DATA_BLOCK "FDB_DP_CMD"
TITLE =
VERSION : 0.1
NON_RETAIN


  STRUCT
   cPLC_OK : BOOL ;	//Trvale Log.1 - test komunikace s PLC
   cBLOKADY_OK : BOOL ;	//Splnìny blokády provozu kotle
   cHORI_UHLI : BOOL ;	//Provoz uhelných hoøákù
   Bit0_03 : BOOL ;
   Bit0_04 : BOOL ;
   Bit0_05 : BOOL ;
   Bit0_06 : BOOL ;
   cACK_ALL : BOOL ;	//Kvitace celková pro všechny hoøáky
   cSTART_H1 : BOOL ;	//Start/Stop hoøáku H1
   Bit1_01 : BOOL ;
   Bit1_02 : BOOL ;
   Bit1_03 : BOOL ;
   Bit1_04 : BOOL ;
   Bit1_05 : BOOL ;
   Bit1_06 : BOOL ;
   cACK_H1 : BOOL ;	//Kvitace hoøáku H1
   cSTART_H2 : BOOL ;	//Start/Stop hoøáku H2
   Bit2_01 : BOOL ;
   Bit2_02 : BOOL ;
   Bit2_03 : BOOL ;
   Bit2_04 : BOOL ;
   Bit2_05 : BOOL ;
   Bit2_06 : BOOL ;
   cACK_H2 : BOOL ;	//Kvitace hoøáku H2
   cSTART_H3 : BOOL ;	//Start/Stop hoøáku H3
   Bit3_01 : BOOL ;
   Bit3_02 : BOOL ;
   Bit3_03 : BOOL ;
   Bit3_04 : BOOL ;
   Bit3_05 : BOOL ;
   Bit3_06 : BOOL ;
   cACK_H3 : BOOL ;	//Kvitace hoøáku H2
   cSTART_H4 : BOOL ;	//Start/Stop hoøáku H4
   Bit4_01 : BOOL ;
   Bit4_02 : BOOL ;
   Bit4_03 : BOOL ;
   Bit4_04 : BOOL ;
   Bit4_05 : BOOL ;
   Bit4_06 : BOOL ;
   cACK_H4 : BOOL ;	//Kvitace hoøáku H4
   W6 : WORD ;
   cSP_H1 : INT ;	//Žádaný výkon hoøáku H1 [0..10000]=[0..100%]
   cSP_H2 : INT ;	//Žádaný výkon hoøáku H2 [0..10000]=[0..100%]
   cSP_H3 : INT ;	//Žádaný výkon hoøáku H3 [0..10000]=[0..100%]
   cSP_H4 : INT ;	//Žádaný výkon hoøáku H4 [0..10000]=[0..100%]
  END_STRUCT ;
BEGIN
   cPLC_OK := FALSE;
   cBLOKADY_OK := FALSE;
   cHORI_UHLI := FALSE;
   Bit0_03 := FALSE;
   Bit0_04 := FALSE;
   Bit0_05 := FALSE;
   Bit0_06 := FALSE;
   cACK_ALL := FALSE;
   cSTART_H1 := FALSE;
   Bit1_01 := FALSE;
   Bit1_02 := FALSE;
   Bit1_03 := FALSE;
   Bit1_04 := FALSE;
   Bit1_05 := FALSE;
   Bit1_06 := FALSE;
   cACK_H1 := FALSE;
   cSTART_H2 := FALSE;
   Bit2_01 := FALSE;
   Bit2_02 := FALSE;
   Bit2_03 := FALSE;
   Bit2_04 := FALSE;
   Bit2_05 := FALSE;
   Bit2_06 := FALSE;
   cACK_H2 := FALSE;
   cSTART_H3 := FALSE;
   Bit3_01 := FALSE;
   Bit3_02 := FALSE;
   Bit3_03 := FALSE;
   Bit3_04 := FALSE;
   Bit3_05 := FALSE;
   Bit3_06 := FALSE;
   cACK_H3 := FALSE;
   cSTART_H4 := FALSE;
   Bit4_01 := FALSE;
   Bit4_02 := FALSE;
   Bit4_03 := FALSE;
   Bit4_04 := FALSE;
   Bit4_05 := FALSE;
   Bit4_06 := FALSE;
   cACK_H4 := FALSE;
   W6 := W#16#0;
   cSP_H1 := 0;
   cSP_H2 := 0;
   cSP_H3 := 0;
   cSP_H4 := 0;
END_DATA_BLOCK

DATA_BLOCK "FDB_DP_STATE"
TITLE =
VERSION : 0.1
NON_RETAIN


  STRUCT
   sPLC_OK : BOOL ;	//Trvale Log.1 - test komunikace s PLC
   sSYSTEM_OK : BOOL ;	//Systém pøipraven (STOP tl., napájení, HW)
   Bit0_02 : BOOL ;
   Bit0_03 : BOOL ;
   sERROR_Hx : BOOL ;	//Spoleèná porucha hoøákù (technologická)
   sSAFE_ERR : BOOL ;	//Porucha SAFETY I/O PLC
   Bit0_06 : BOOL ;
   sACK_REQ : BOOL ;	//Systém vyžaduje kvitaci
   sPROVOZ_H1 : BOOL ;	//Provoz hoøáku H1
   sREADY_H1 : BOOL ;	//Hoøák pøipraven H1 (STOP tl., napájení, HW)
   sSTART_H1 : BOOL ;	//Start hoøáku H1
   sLOCAL_H1 : BOOL ;	//Lokální øízení hoøáku H1
   sERROR_H1 : BOOL ;	//Porucha hoøáku H1 (technologická)
   sFERR_H1 : BOOL ;	//Porucha SAFETY I/O hoøáku H1
   Bit1_06 : BOOL ;
   sACK_REQ_H1 : BOOL ;	//Hoøák H1 vyžaduje kvitaci
   sPROVOZ_H2 : BOOL ;	//Provoz hoøáku H2
   sREADY_H2 : BOOL ;	//Hoøák pøipraven H2 (STOP tl., napájení, HW)
   sSTART_H2 : BOOL ;	//Start hoøáku H2
   sLOCAL_H2 : BOOL ;	//Lokální øízení hoøáku H2
   sERROR_H2 : BOOL ;	//Porucha hoøáku H2 (technologická)
   sFERR_H2 : BOOL ;	//Porucha SAFETY I/O hoøáku H2
   Bit2_06 : BOOL ;
   sACK_REQ_H2 : BOOL ;	//Hoøák H2 vyžaduje kvitaci
   sPROVOZ_H3 : BOOL ;	//Provoz hoøáku H3
   sREADY_H3 : BOOL ;	//Hoøák pøipraven H3 (STOP tl., napájení, HW)
   sSTART_H3 : BOOL ;	//Start hoøáku H3
   sLOCAL_H3 : BOOL ;	//Lokální øízení hoøáku H3
   sERROR_H3 : BOOL ;	//Porucha hoøáku H3 (technologická)
   sFERR_H3 : BOOL ;	//Porucha SAFETY I/O hoøáku H3
   Bit3_06 : BOOL ;
   sACK_REQ_H3 : BOOL ;	//Hoøák H3 vyžaduje kvitaci
   sPROVOZ_H4 : BOOL ;	//Provoz hoøáku H4
   sREADY_H4 : BOOL ;	//Hoøák pøipraven H4 (STOP tl., napájení, HW)
   sSTART_H4 : BOOL ;	//Start hoøáku H4
   sLOCAL_H4 : BOOL ;	//Lokální øízení hoøáku H4
   sERROR_H4 : BOOL ;	//Porucha hoøáku H4 (technologická)
   sFERR_H4 : BOOL ;	//Porucha SAFETY I/O hoøáku H4
   Bit4_06 : BOOL ;
   sACK_REQ_H4 : BOOL ;	//Hoøák H4 vyžaduje kvitaci
   W6 : WORD ;
   sSP_H1 : INT ;	//Výkon hoøáku H1 [0..10000]=[0..100%]
   sSP_H2 : INT ;	//Výkon hoøáku H2 [0..10000]=[0..100%]
   sSP_H3 : INT ;	//Výkon hoøáku H3 [0..10000]=[0..100%]
   sSP_H4 : INT ;	//Výkon hoøáku H4 [0..10000]=[0..100%]
   K04HJA10CR001XB01 : BOOL ;	//I0.0: HOØÁK È.1 - HLÍDAÈ PLAMENE - PLAMEN HOØÍ
   K04HJA20CR001XB01 : BOOL ;	//I0.1: HOØÁK È.2 - HLÍDAÈ PLAMENE - PLAMEN HOØÍ
   K04HJA30CR001XB01 : BOOL ;	//I0.2: HOØÁK È.3 - HLÍDAÈ PLAMENE - PLAMEN HOØÍ
   K04HJA40CR001XB01 : BOOL ;	//I0.3: HOØÁK È.4 - HLÍDAÈ PLAMENE - PLAMEN HOØÍ
   K04CJF21EA001XB01 : BOOL ;	//I0.4: NAPÁJENÍ HOØÁKU È.1 - OK
   K04CJF21EA001XB02 : BOOL ;	//I0.5: NAPÁJENÍ SERVOPOHONÙ HOØÁK 1 - OK
   K04HHA20AV11XG10 : BOOL ;	//I0.6: HOØÁK È.1 - STYKAÈE BEZP. VYPNUTÍ ROZEPNUTY (PØIPRAVENY)
   K04CJF21EA001XB03 : BOOL ;	//I0.7: NAPÁJENÍ HOØÁKU È.2 - OK
   K04CJF21EA001XB04 : BOOL ;	//I1.0: NAPÁJENÍ SERVOPOHONÙ HOØÁK 2 - OK
   K04HHA20AV21XG10 : BOOL ;	//I1.1: HOØÁK È.2 - STYKAÈE BEZP. VYPNUTÍ ROZEPNUTY (PØIPRAVENY)
   K04CJF21EA001XB05 : BOOL ;	//I1.2: NAPÁJENÍ HOØÁKU È.3 - OK
   K04CJF21EA001XB06 : BOOL ;	//I1.3: NAPÁJENÍ SERVOPOHONÙ HOØÁK 3 - OK
   K04HHA20AV31XG10 : BOOL ;	//I1.4: HOØÁK È.3 - STYKAÈE BEZP. VYPNUTÍ ROZEPNUTY (PØIPRAVENY)
   K04CJF21EA001XB07 : BOOL ;	//I1.5: NAPÁJENÍ HOØÁKU È.4 - OK
   K04CJF21EA001XB08 : BOOL ;	//I1.6: NAPÁJENÍ SERVOPOHONÙ HOØÁK 4 - OK
   K04HHA20AV41XG10 : BOOL ;	//I1.7: HOØÁK È.3 - STYKAÈE BEZP. VYPNUTÍ ROZEPNUTY (PØIPRAVENY)
   K04HJA10CR001XB51 : BOOL ;	//I100.0: HOØÁK È.1 - PLAMEN HOØÍ HLÍDAÈ PLAMENE (FAIL SAFE)
   K04HJA20CR001XB51 : BOOL ;	//I100.1: HOØÁK È.2 - PLAMEN HOØÍ HLÍDAÈ PLAMENE (FAIL SAFE)
   K04HJA30CR001XB51 : BOOL ;	//I100.2: HOØÁK È.3 - PLAMEN HOØÍ HLÍDAÈ PLAMENE (FAIL SAFE)
   K04HJA40CR001XB51 : BOOL ;	//I100.3: HOØÁK È.4 - PLAMEN HOØÍ HLÍDAÈ PLAMENE (FAIL SAFE)
   K04HHG36CP031XG01 : BOOL ;	//I100.4: HOØÁK 1 - TLAK PLYNU MIN - ZKOUŠKA TÌSNOSTI
   K04HHL11CP001XG01 : BOOL ;	//I100.5: HOØÁK 1 - TLAK SEKUNDÁRNÍHO VZDUCHU MIN
   K04HHA20AV011XB01 : BOOL ;	//I100.6: HOØÁK 1 - HOØÁK - ZAPALOVACÍ PLAMEN
   K04HHG37CP031XG01 : BOOL ;	//I100.7: HOØÁK 2 - TLAK PLYNU MIN - ZKOUŠKA TÌSNOSTI
   K04HHL71CP001XG01 : BOOL ;	//I101.0: HOØÁK 2 - TLAK SEKUNDÁRNÍHO VZDUCHU MIN
   K04HHA20AV021XB01 : BOOL ;	//I101.1: HOØÁK 2 - HOØÁK - ZAPALOVACÍ PLAMEN
   K04HHG38CP031XG01 : BOOL ;	//I101.2: HOØÁK 3 - TLAK PLYNU MIN - ZKOUŠKA TÌSNOSTI
   K04HHL51CP001XG01 : BOOL ;	//I101.3: HOØÁK 3 - TLAK SEKUNDÁRNÍHO VZDUCHU MIN
   K04HHA20AV031XB01 : BOOL ;	//I101.4: HOØÁK 3 - HOØÁK - ZAPALOVACÍ PLAMEN
   K04HHG39CP031XG01 : BOOL ;	//I101.5: HOØÁK 4 - TLAK PLYNU MIN - ZKOUŠKA TÌSNOSTI
   K04HHL31CP001XG01 : BOOL ;	//I101.6: HOØÁK 4 - TLAK SEKUNDÁRNÍHO VZDUCHU MIN
   K04HHA20AV041XB01 : BOOL ;	//I101.7: HOØÁK 4 - HOØÁK - ZAPALOVACÍ PLAMEN
   K04HHL11AS010XB51 : BOOL ;	//I102.0: HOØÁK È.1 - POLOHA KLAPKY VZDUCHU PRO ZAPALOVÁNÍ
   K04HHL11AS010XB53 : BOOL ;	//I102.1: HOØÁK È.1 - POLOHA KLAPKY VZDUCHU PRO PROFUK
   K04HHG36AS001XB51 : BOOL ;	//I102.2: HOØÁK È.1 - POLOHA KLAPKY PLYNU PRO ZAPALOVÁNÍ
   K04HHL71AS010XB51 : BOOL ;	//I102.3: HOØÁK È.2 - POLOHA KLAPKY VZDUCHU PRO ZAPALOVÁNÍ
   K04HHL71AS010XB53 : BOOL ;	//I102.4: HOØÁK È.2 - POLOHA KLAPKY VZDUCHU PRO PROFUK
   K04HHG37AS001XB51 : BOOL ;	//I102.5: HOØÁK È.2 - POLOHA KLAPKY PLYNU PRO ZAPALOVÁNÍ
   K04HHL51AS010XB51 : BOOL ;	//I102.6: HOØÁK È.3 - POLOHA KLAPKY VZDUCHU PRO ZAPALOVÁNÍ
   K04HHL51AS010XB53 : BOOL ;	//I102.7: HOØÁK È.3 - POLOHA KLAPKY VZDUCHU PRO PROFUK
   K04HHG38AS001XB51 : BOOL ;	//I110.0: HOØÁK È.3 - POLOHA KLAPKY PLYNU PRO ZAPALOVÁNÍ
   K04HHL31AS010XB51 : BOOL ;	//I110.1: HOØÁK È.4 - POLOHA KLAPKY VZDUCHU PRO ZAPALOVÁNÍ
   K04HHL31AS010XB53 : BOOL ;	//I110.2: HOØÁK È.4 - POLOHA KLAPKY VZDUCHU PRO PROFUK
   K04HHG39AS001XB51 : BOOL ;	//I110.3: HOØÁK È.4 - POLOHA KLAPKY PLYNU PRO ZAPALOVÁNÍ
   K04HHA20CH001YG11 : BOOL ;	//I110.4: TLAÈÍTKO BEZPEÈNOSTNÍ VYPNUTÍ - DVEØE ROZVADÌÈE
   K04HHA20CH001YG21 : BOOL ;	//I110.5: TLAÈÍTKO BEZPEÈNOSTNÍ VYPNUTÍ - OVLÁDACÍ SKØÍÒKA
   K04HHA20CH001YG31 : BOOL ;	//I110.6: TLAÈÍTKO BEZPEÈNOSTNÍ VYPNUTÍ - TLAÈÍTKO U DVEØÍ
   FI110_7 : BOOL ;	//I110.7: REZERVA
   K04HHG36CP001XG01 : BOOL ;	//I111.0: HOØÁK 1 - TLAK PLYNU MIN
   K04HHG36CP002XG01 : BOOL ;	//I111.1: HOØÁK 1 - TLAK PLYNU MAX
   K04HHG37CP001XG01 : BOOL ;	//I111.2: HOØÁK 2 - TLAK PLYNU MIN
   K04HHG37CP002XG01 : BOOL ;	//I111.3: HOØÁK 2 - TLAK PLYNU MAX
   K04HHG38CP001XG01 : BOOL ;	//I111.4: HOØÁK 3 - TLAK PLYNU MIN
   K04HHG38CP002XG01 : BOOL ;	//I111.5: HOØÁK 3 - TLAK PLYNU MAX
   K04HHG39CP001XG01 : BOOL ;	//I111.6: HOØÁK 4 - TLAK PLYNU MIN
   K04HHG39CP002XG01 : BOOL ;	//I111.7: HOØÁK 4 - TLAK PLYNU MAX
   FI112_0 : BOOL ;	//I112.0: REZERVA
   FI112_1 : BOOL ;	//I112.1: REZERVA
   FI112_2 : BOOL ;	//I112.2: REZERVA
   FI112_3 : BOOL ;	//I112.3: REZERVA
   FI112_4 : BOOL ;	//I112.4: REZERVA
   FI112_5 : BOOL ;	//I112.5: REZERVA
   FI112_6 : BOOL ;	//I112.6: REZERVA
   FI112_7 : BOOL ;	//I112.7: REZERVA
   K04HJA10CR001YB01 : BOOL ;	//Q0.0: HOØÁK 1 - UVOLNÌNÍ SNÍMAÈE PLAMENE
   K04HHL11AA101YB01 : BOOL ;	//Q0.1: HOØÁK 1 - TØÍCESTNÝ VENTIL SPAL. VZDUCHU - OTEVØÍT
   K04HJA20CR001YB01 : BOOL ;	//Q0.2: HOØÁK 2 - UVOLNÌNÍ SNÍMAÈE PLAMENE
   K04HHL71AA101YB01 : BOOL ;	//Q0.3: HOØÁK 2 - TØÍCESTNÝ VENTIL SPAL. VZDUCHU - OTEVØÍT
   K04HJA30CR001YB01 : BOOL ;	//Q0.4: HOØÁK 3 - UVOLNÌNÍ SNÍMAÈE PLAMENE
   K04HHL51AA101YB01 : BOOL ;	//Q0.5: HOØÁK 3 - TØÍCESTNÝ VENTIL SPAL. VZDUCHU - OTEVØÍT
   K04HJA40CR001YB01 : BOOL ;	//Q0.6: HOØÁK 4 - UVOLNÌNÍ SNÍMAÈE PLAMENE
   K04HHL31AA101YB01 : BOOL ;	//Q0.7: HOØÁK 4 - TØÍCESTNÝ VENTIL SPAL. VZDUCHU - OTEVØÍT
   Q1_0 : BOOL ;	//Q1.0: REZERVA
   Q1_1 : BOOL ;	//Q1.1: REZERVA
   Q1_2 : BOOL ;	//Q1.2: REZERVA
   Q1_3 : BOOL ;	//Q1.3: REZERVA
   Q1_4 : BOOL ;	//Q1.4: REZERVA
   Q1_5 : BOOL ;	//Q1.5: REZERVA
   Q1_6 : BOOL ;	//Q1.6: REZERVA
   Q1_7 : BOOL ;	//Q1.7: REZERVA
   K04HHA20AV011YB03 : BOOL ;	//Q200.0: VYPNUTÍ HOØÁKU 1 - FAIL SAFE
   K04HHG36AA101YB01 : BOOL ;	//Q200.1: HOØÁK 1 - PRVNÍ VENTIL PALIVA - OTEVØÍT
   K04HHG36AA102YB01 : BOOL ;	//Q200.2: HOØÁK 1 - DRUHÝ VENTIL PALIVA - OTEVØÍT
   K04HHG36AA131YB01 : BOOL ;	//Q200.3: HOØÁK 1 - ODVZDUŠÒOVACÍ VENTIL - OTEVØÍT
   K04HJA10AA101YB01 : BOOL ;	//Q200.4: HOØÁK 1 - SOL.UZÁVÌR PØÍVODU PLYNU ZAP.HOØÁKU - OTEVØÍT
   K04HHA20AV021YB03 : BOOL ;	//Q200.5: VYPNUTÍ HOØÁKU 2 - FAIL SAFE
   K04HHG37AA101YB01 : BOOL ;	//Q200.6: HOØÁK 2 - PRVNÍ VENTIL PALIVA - OTEVØÍT
   K04HHG37AA102YB01 : BOOL ;	//Q200.7: HOØÁK 2 - DRUHÝ VENTIL PALIVA - OTEVØÍT
   K04HHG37AA131YB01 : BOOL ;	//Q201.0: HOØÁK 2 - ODVZDUŠÒOVACÍ VENTIL - OTEVØÍT
   K04HJA20AA101YB01 : BOOL ;	//Q201.1: HOØÁK 2 - SOL.UZÁVÌR PØÍVODU PLYNU ZAP.HOØÁKU - OTEVØÍT
   FQ201_2 : BOOL ;	//REZERVA
   FQ201_3 : BOOL ;	//REZERVA
   FQ201_4 : BOOL ;	//REZERVA
   FQ201_5 : BOOL ;	//REZERVA
   FQ201_6 : BOOL ;	//REZERVA
   FQ201_7 : BOOL ;	//REZERVA
   K04HHA20AV031YB03 : BOOL ;	//Q208.0: VYPNUTÍ HOØÁKU 3 - FAIL SAFE
   K04HHG38AA101YB01 : BOOL ;	//Q208.1: HOØÁK 3 - PRVNÍ VENTIL PALIVA - OTEVØÍT
   K04HHG38AA102YB01 : BOOL ;	//Q208.2: HOØÁK 3 - DRUHÝ VENTIL PALIVA - OTEVØÍT
   K04HHG38AA131YB01 : BOOL ;	//Q208.3: HOØÁK 3 - ODVZDUŠÒOVACÍ VENTIL - OTEVØÍT
   K04HJA30AA101YB01 : BOOL ;	//Q208.4: HOØÁK 3 - SOL.UZÁVÌR PØÍVODU PLYNU ZAP.HOØÁKU - OTEVØÍT
   K04HHA20AV041YB03 : BOOL ;	//Q208.5: VYPNUTÍ HOØÁKU 4 - FAIL SAFE
   K04HHG39AA101YB01 : BOOL ;	//Q208.6: HOØÁK 4 - PRVNÍ VENTIL PALIVA - OTEVØÍT
   K04HHG39AA102YB01 : BOOL ;	//Q208.7: HOØÁK 4 - DRUHÝ VENTIL PALIVA - OTEVØÍT
   K04HHG39AA131YB01 : BOOL ;	//Q209.0: HOØÁK 4 - ODVZDUŠÒOVACÍ VENTIL - OTEVØÍT
   K04HJA40AA101YB01 : BOOL ;	//Q209.1: HOØÁK 4 - SOL.UZÁVÌR PØÍVODU PLYNU ZAP.HOØÁKU - OTEVØÍT
   FQ209_2 : BOOL ;	//REZERVA
   FQ209_3 : BOOL ;	//REZERVA
   FQ209_4 : BOOL ;	//REZERVA
   FQ209_5 : BOOL ;	//REZERVA
   FQ209_6 : BOOL ;	//REZERVA
   FQ209_7 : BOOL ;	//REZERVA
   K04HHA20AV11YB01 : BOOL ;	//Q216.0: HOØÁK 1 - ZAPALOVAÈ
   K04HHA20AV21YB01 : BOOL ;	//Q216.1: HOØÁK 2 - ZAPALOVAÈ
   K04HHA20AV31YB01 : BOOL ;	//Q216.2: HOØÁK 3 - ZAPALOVAÈ
   K04HHA20AV41YB01 : BOOL ;	//Q216.3: HOØÁK 4 - ZAPALOVAÈ
   FQ216_4 : BOOL ;	//Q216.4: REZERVA
   FQ216_5 : BOOL ;	//Q216.5: REZERVA
   FQ216_6 : BOOL ;	//Q216.6: REZERVA
   FQ216_7 : BOOL ;	//Q216.7: REZERVA
   FQ217_0 : BOOL ;	//Q217.0: REZERVA
   FQ217_1 : BOOL ;	//Q217.1: REZERVA
   K04HJA10CR001XQ01 : WORD ;	//PIW512: HOØÁK È.1 - VELIKOST PLAMENE 4-20mA
   K04HJA20CR001XQ01 : WORD ;	//PIW514: HOØÁK È.2 - VELIKOST PLAMENE 4-20mA
   K04HJA30CR001XQ01 : WORD ;	//PIW516: HOØÁK È.3 - VELIKOST PLAMENE 4-20mA
   K04HJA40CR001XQ01 : WORD ;	//PIW518: HOØÁK È.4 - VELIKOST PLAMENE 4-20mA
   K04HHG36AS001XQ01 : WORD ;	//PIW520: HOØÁK È.1 - POLOHA KLAPKY PLYNU
   K04HHL11AS010XQ01 : WORD ;	//PIW522: HOØÁK È.1 - POLOHA KLAPKY VZDUCHU
   K04HHG37AS001XQ01 : WORD ;	//PIW524: HOØÁK È.2 - POLOHA KLAPKY PLYNU
   K04HHL71AS010XQ01 : WORD ;	//PIW526: HOØÁK È.2 - POLOHA KLAPKY VZDUCHU
   K04HHG38AS001XQ01 : WORD ;	//PIW528: HOØÁK È.3 - POLOHA KLAPKY PLYNU
   K04HHL51AS010XQ01 : WORD ;	//PIW530: HOØÁK È.3 - POLOHA KLAPKY VZDUCHU
   K04HHG39AS001XQ01 : WORD ;	//PIW532: HOØÁK È.4 - POLOHA KLAPKY PLYNU
   K04HHL31AS010XQ01 : WORD ;	//PIW534: HOØÁK È.4 - POLOHA KLAPKY VZDUCHU
   GAS_BU_STATUS_H1 : INT ;	//Ovládání hoøáku H1 - STATUS
   GAS_BU_DIAG_H1 : WORD ;	//Ovládání hoøáku H1 - DIAGNOSTIKA
   TIGHTN_STATUS_H1 : INT ;	//Test tìsnosti H1 - STATUS
   TIGHTN_DIAG_H1 : WORD ;	//Test tìsnosti H1 - DIAGNOSTIKA
   IGNTR_STATUS_H1 : INT ;	//Zapalovací hoøák H1 - STATUS
   IGNTR_DIAG_H1 : WORD ;	//Zapalovací hoøák H1 - DIAGNOSTIKA
   PREPURGE_STATUS_H1 : INT ;	//Provìtrávání H1 - STATUS
   PREPURGE_DIAG_H1 : WORD ;	//Provìtrávání H1 - DIAGNOSTIKA
   VALVE_DIAG_H1 : WORD ;	//Regulaèní klapky H1 - DIAGNOSTIKA
   GAS_BU_STATUS_H2 : INT ;	//Ovládání hoøáku H2 - STATUS
   GAS_BU_DIAG_H2 : WORD ;	//Ovládání hoøáku H2 - DIAGNOSTIKA
   TIGHTN_STATUS_H2 : INT ;	//Test tìsnosti H2 - STATUS
   TIGHTN_DIAG_H2 : WORD ;	//Test tìsnosti H2 - DIAGNOSTIKA
   IGNTR_STATUS_H2 : INT ;	//Zapalovací hoøák H2 - STATUS
   IGNTR_DIAG_H2 : WORD ;	//Zapalovací hoøák H2 - DIAGNOSTIKA
   PREPURGE_STATUS_H2 : INT ;	//Provìtrávání H2 - STATUS
   PREPURGE_DIAG_H2 : WORD ;	//Provìtrávání H2 - DIAGNOSTIKA
   VALVE_DIAG_H2 : WORD ;	//Regulaèní klapky H2 - DIAGNOSTIKA
   GAS_BU_STATUS_H3 : INT ;	//Ovládání hoøáku H3 - STATUS
   GAS_BU_DIAG_H3 : WORD ;	//Ovládání hoøáku H3 - DIAGNOSTIKA
   TIGHTN_STATUS_H3 : INT ;	//Test tìsnosti H3 - STATUS
   TIGHTN_DIAG_H3 : WORD ;	//Test tìsnosti H3 - DIAGNOSTIKA
   IGNTR_STATUS_H3 : INT ;	//Zapalovací hoøák H3 - STATUS
   IGNTR_DIAG_H3 : WORD ;	//Zapalovací hoøák H3 - DIAGNOSTIKA
   PREPURGE_STATUS_H3 : INT ;	//Provìtrávání H3 - STATUS
   PREPURGE_DIAG_H3 : WORD ;	//Provìtrávání H3 - DIAGNOSTIKA
   VALVE_DIAG_H3 : WORD ;	//Regulaèní klapky H3 - DIAGNOSTIKA
   GAS_BU_STATUS_H4 : INT ;	//Ovládání hoøáku H4 - STATUS
   GAS_BU_DIAG_H4 : WORD ;	//Ovládání hoøáku H4 - DIAGNOSTIKA
   TIGHTN_STATUS_H4 : INT ;	//Test tìsnosti H4 - STATUS
   TIGHTN_DIAG_H4 : WORD ;	//Test tìsnosti H4 - DIAGNOSTIKA
   IGNTR_STATUS_H4 : INT ;	//Zapalovací hoøák H4 - STATUS
   IGNTR_DIAG_H4 : WORD ;	//Zapalovací hoøák H4 - DIAGNOSTIKA
   PREPURGE_STATUS_H4 : INT ;	//Provìtrávání H4 - STATUS
   PREPURGE_DIAG_H4 : WORD ;	//Provìtrávání H4 - DIAGNOSTIKA
   VALVE_DIAG_H4 : WORD ;	//Regulaèní klapky H4 - DIAGNOSTIKA
  END_STRUCT ;
BEGIN
   sPLC_OK := FALSE;
   sSYSTEM_OK := FALSE;
   Bit0_02 := FALSE;
   Bit0_03 := FALSE;
   sERROR_Hx := FALSE;
   sSAFE_ERR := FALSE;
   Bit0_06 := FALSE;
   sACK_REQ := FALSE;
   sPROVOZ_H1 := FALSE;
   sREADY_H1 := FALSE;
   sSTART_H1 := FALSE;
   sLOCAL_H1 := FALSE;
   sERROR_H1 := FALSE;
   sFERR_H1 := FALSE;
   Bit1_06 := FALSE;
   sACK_REQ_H1 := FALSE;
   sPROVOZ_H2 := FALSE;
   sREADY_H2 := FALSE;
   sSTART_H2 := FALSE;
   sLOCAL_H2 := FALSE;
   sERROR_H2 := FALSE;
   sFERR_H2 := FALSE;
   Bit2_06 := FALSE;
   sACK_REQ_H2 := FALSE;
   sPROVOZ_H3 := FALSE;
   sREADY_H3 := FALSE;
   sSTART_H3 := FALSE;
   sLOCAL_H3 := FALSE;
   sERROR_H3 := FALSE;
   sFERR_H3 := FALSE;
   Bit3_06 := FALSE;
   sACK_REQ_H3 := FALSE;
   sPROVOZ_H4 := FALSE;
   sREADY_H4 := FALSE;
   sSTART_H4 := FALSE;
   sLOCAL_H4 := FALSE;
   sERROR_H4 := FALSE;
   sFERR_H4 := FALSE;
   Bit4_06 := FALSE;
   sACK_REQ_H4 := FALSE;
   W6 := W#16#0;
   sSP_H1 := 0;
   sSP_H2 := 0;
   sSP_H3 := 0;
   sSP_H4 := 0;
   K04HJA10CR001XB01 := FALSE;
   K04HJA20CR001XB01 := FALSE;
   K04HJA30CR001XB01 := FALSE;
   K04HJA40CR001XB01 := FALSE;
   K04CJF21EA001XB01 := FALSE;
   K04CJF21EA001XB02 := FALSE;
   K04HHA20AV11XG10 := FALSE;
   K04CJF21EA001XB03 := FALSE;
   K04CJF21EA001XB04 := FALSE;
   K04HHA20AV21XG10 := FALSE;
   K04CJF21EA001XB05 := FALSE;
   K04CJF21EA001XB06 := FALSE;
   K04HHA20AV31XG10 := FALSE;
   K04CJF21EA001XB07 := FALSE;
   K04CJF21EA001XB08 := FALSE;
   K04HHA20AV41XG10 := FALSE;
   K04HJA10CR001XB51 := FALSE;
   K04HJA20CR001XB51 := FALSE;
   K04HJA30CR001XB51 := FALSE;
   K04HJA40CR001XB51 := FALSE;
   K04HHG36CP031XG01 := FALSE;
   K04HHL11CP001XG01 := FALSE;
   K04HHA20AV011XB01 := FALSE;
   K04HHG37CP031XG01 := FALSE;
   K04HHL71CP001XG01 := FALSE;
   K04HHA20AV021XB01 := FALSE;
   K04HHG38CP031XG01 := FALSE;
   K04HHL51CP001XG01 := FALSE;
   K04HHA20AV031XB01 := FALSE;
   K04HHG39CP031XG01 := FALSE;
   K04HHL31CP001XG01 := FALSE;
   K04HHA20AV041XB01 := FALSE;
   K04HHL11AS010XB51 := FALSE;
   K04HHL11AS010XB53 := FALSE;
   K04HHG36AS001XB51 := FALSE;
   K04HHL71AS010XB51 := FALSE;
   K04HHL71AS010XB53 := FALSE;
   K04HHG37AS001XB51 := FALSE;
   K04HHL51AS010XB51 := FALSE;
   K04HHL51AS010XB53 := FALSE;
   K04HHG38AS001XB51 := FALSE;
   K04HHL31AS010XB51 := FALSE;
   K04HHL31AS010XB53 := FALSE;
   K04HHG39AS001XB51 := FALSE;
   K04HHA20CH001YG11 := FALSE;
   K04HHA20CH001YG21 := FALSE;
   K04HHA20CH001YG31 := FALSE;
   FI110_7 := FALSE;
   K04HHG36CP001XG01 := FALSE;
   K04HHG36CP002XG01 := FALSE;
   K04HHG37CP001XG01 := FALSE;
   K04HHG37CP002XG01 := FALSE;
   K04HHG38CP001XG01 := FALSE;
   K04HHG38CP002XG01 := FALSE;
   K04HHG39CP001XG01 := FALSE;
   K04HHG39CP002XG01 := FALSE;
   FI112_0 := FALSE;
   FI112_1 := FALSE;
   FI112_2 := FALSE;
   FI112_3 := FALSE;
   FI112_4 := FALSE;
   FI112_5 := FALSE;
   FI112_6 := FALSE;
   FI112_7 := FALSE;
   K04HJA10CR001YB01 := FALSE;
   K04HHL11AA101YB01 := FALSE;
   K04HJA20CR001YB01 := FALSE;
   K04HHL71AA101YB01 := FALSE;
   K04HJA30CR001YB01 := FALSE;
   K04HHL51AA101YB01 := FALSE;
   K04HJA40CR001YB01 := FALSE;
   K04HHL31AA101YB01 := FALSE;
   Q1_0 := FALSE;
   Q1_1 := FALSE;
   Q1_2 := FALSE;
   Q1_3 := FALSE;
   Q1_4 := FALSE;
   Q1_5 := FALSE;
   Q1_6 := FALSE;
   Q1_7 := FALSE;
   K04HHA20AV011YB03 := FALSE;
   K04HHG36AA101YB01 := FALSE;
   K04HHG36AA102YB01 := FALSE;
   K04HHG36AA131YB01 := FALSE;
   K04HJA10AA101YB01 := FALSE;
   K04HHA20AV021YB03 := FALSE;
   K04HHG37AA101YB01 := FALSE;
   K04HHG37AA102YB01 := FALSE;
   K04HHG37AA131YB01 := FALSE;
   K04HJA20AA101YB01 := FALSE;
   FQ201_2 := FALSE;
   FQ201_3 := FALSE;
   FQ201_4 := FALSE;
   FQ201_5 := FALSE;
   FQ201_6 := FALSE;
   FQ201_7 := FALSE;
   K04HHA20AV031YB03 := FALSE;
   K04HHG38AA101YB01 := FALSE;
   K04HHG38AA102YB01 := FALSE;
   K04HHG38AA131YB01 := FALSE;
   K04HJA30AA101YB01 := FALSE;
   K04HHA20AV041YB03 := FALSE;
   K04HHG39AA101YB01 := FALSE;
   K04HHG39AA102YB01 := FALSE;
   K04HHG39AA131YB01 := FALSE;
   K04HJA40AA101YB01 := FALSE;
   FQ209_2 := FALSE;
   FQ209_3 := FALSE;
   FQ209_4 := FALSE;
   FQ209_5 := FALSE;
   FQ209_6 := FALSE;
   FQ209_7 := FALSE;
   K04HHA20AV11YB01 := FALSE;
   K04HHA20AV21YB01 := FALSE;
   K04HHA20AV31YB01 := FALSE;
   K04HHA20AV41YB01 := FALSE;
   FQ216_4 := FALSE;
   FQ216_5 := FALSE;
   FQ216_6 := FALSE;
   FQ216_7 := FALSE;
   FQ217_0 := FALSE;
   FQ217_1 := FALSE;
   K04HJA10CR001XQ01 := W#16#0;
   K04HJA20CR001XQ01 := W#16#0;
   K04HJA30CR001XQ01 := W#16#0;
   K04HJA40CR001XQ01 := W#16#0;
   K04HHG36AS001XQ01 := W#16#0;
   K04HHL11AS010XQ01 := W#16#0;
   K04HHG37AS001XQ01 := W#16#0;
   K04HHL71AS010XQ01 := W#16#0;
   K04HHG38AS001XQ01 := W#16#0;
   K04HHL51AS010XQ01 := W#16#0;
   K04HHG39AS001XQ01 := W#16#0;
   K04HHL31AS010XQ01 := W#16#0;
   GAS_BU_STATUS_H1 := 0;
   GAS_BU_DIAG_H1 := W#16#0;
   TIGHTN_STATUS_H1 := 0;
   TIGHTN_DIAG_H1 := W#16#0;
   IGNTR_STATUS_H1 := 0;
   IGNTR_DIAG_H1 := W#16#0;
   PREPURGE_STATUS_H1 := 0;
   PREPURGE_DIAG_H1 := W#16#0;
   VALVE_DIAG_H1 := W#16#0;
   GAS_BU_STATUS_H2 := 0;
   GAS_BU_DIAG_H2 := W#16#0;
   TIGHTN_STATUS_H2 := 0;
   TIGHTN_DIAG_H2 := W#16#0;
   IGNTR_STATUS_H2 := 0;
   IGNTR_DIAG_H2 := W#16#0;
   PREPURGE_STATUS_H2 := 0;
   PREPURGE_DIAG_H2 := W#16#0;
   VALVE_DIAG_H2 := W#16#0;
   GAS_BU_STATUS_H3 := 0;
   GAS_BU_DIAG_H3 := W#16#0;
   TIGHTN_STATUS_H3 := 0;
   TIGHTN_DIAG_H3 := W#16#0;
   IGNTR_STATUS_H3 := 0;
   IGNTR_DIAG_H3 := W#16#0;
   PREPURGE_STATUS_H3 := 0;
   PREPURGE_DIAG_H3 := W#16#0;
   VALVE_DIAG_H3 := W#16#0;
   GAS_BU_STATUS_H4 := 0;
   GAS_BU_DIAG_H4 := W#16#0;
   TIGHTN_STATUS_H4 := 0;
   TIGHTN_DIAG_H4 := W#16#0;
   IGNTR_STATUS_H4 := 0;
   IGNTR_DIAG_H4 := W#16#0;
   PREPURGE_STATUS_H4 := 0;
   PREPURGE_DIAG_H4 := W#16#0;
   VALVE_DIAG_H4 := W#16#0;
END_DATA_BLOCK

